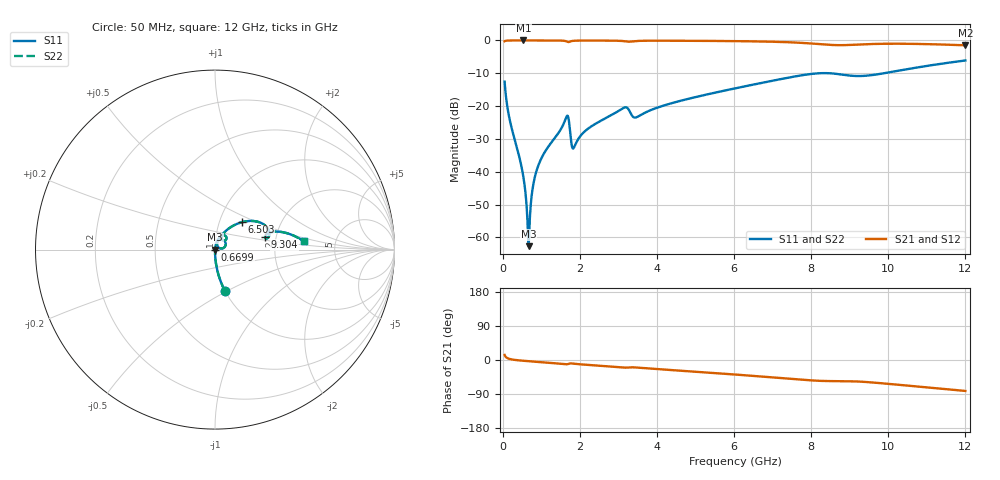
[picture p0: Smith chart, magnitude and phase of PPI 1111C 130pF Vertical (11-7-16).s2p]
# GHz S MA R 50
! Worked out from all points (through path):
!   1601 points, 50 MHz to 12 GHz, reference 50 ohm
!   highest |S21| = -0.01 dB at 535.5 MHz (marker M1); lowest = -1.5 dB at 12 GHz (marker M2)
!   group delay of S21, straight-line fit = 18.7 ps
!   lowest |S11| = -62.7 dB at 669.9 MHz (marker M3), VSWR 1.00, Z = 50.1 - j0.0112 ohm
!   |S11| at or under -10 dB: start of sweep to 8.202 GHz; 8.484 GHz to 9.885 GHz (1.401 GHz wide, 15.3 % of centre)
!   |S22| runs from -62.7 to -6.1 dB; largest |S21 - S12| = 0
!   S11 on the Smith chart (normalised r, x): 50 MHz: 1.00, -0.49; 669.9 MHz: 1.00, -0.00; 6.503 GHz: 1.28, +0.41; 9.304 GHz: 1.75, +0.27; 12 GHz: 2.91, +0.36
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0.05  0.2359 -76.5  0.9715 13.4  0.9715 13.4  0.2359 -76.5
0.1844375  0.06115 -87.0  0.9977 2.6  0.9977 2.6  0.06115 -87.0
0.5354688  0.008428 -87.5  0.9993 -2.0  0.9993 -2.0  0.008428 -87.5
0.6325625  0.002314 -74.9  0.9992 -2.8  0.9992 -2.8  0.002314 -74.9
0.6699063  0.0007361 -8.7  0.9992 -3.1  0.9992 -3.1  0.0007361 -8.7
0.70725  0.002094 65.5  0.9992 -3.4  0.9992 -3.4  0.002094 65.5
0.7744688  0.005451 77.7  0.9991 -4.0  0.9991 -4.0  0.005451 77.7
0.8416875  0.008675 80.1  0.9991 -4.5  0.9991 -4.5  0.008675 80.1
1.103094  0.02045 80.7  0.9987 -6.4  0.9987 -6.4  0.02045 80.7
1.655781  0.06891 52.5  0.9676 -11.3  0.9676 -11.3  0.06891 52.5
1.700594  0.06786 28.1  0.9459 -10.4  0.9459 -10.4  0.06786 28.1
1.827562  0.02258 42.5  0.9859 -9.6  0.9859 -9.6  0.02258 42.5
2.044156  0.03677 72.1  0.9952 -11.7  0.9952 -11.7  0.03677 72.1
3.142063  0.09442 57.7  0.9753 -20.0  0.9753 -20.0  0.09442 57.7
3.440812  0.06687 52.7  0.9775 -19.7  0.9775 -19.7  0.06687 52.7
4.038312  0.09602 63.0  0.9906 -24.3  0.9906 -24.3  0.09602 63.0
6.025  0.1862 49.8  0.9762 -38.3  0.9762 -38.3  0.1862 49.8
6.503  0.2127 45.7  0.9681 -42.0  0.9681 -42.0  0.2127 45.7
8.019156  0.3095 25.8  0.8969 -53.9  0.8969 -53.9  0.3095 25.8
9.303781  0.2874 14.1  0.8697 -57.3  0.8697 -57.3  0.2874 14.1
10.01331  0.3259 17.2  0.891 -63.0  0.891 -63.0  0.3259 17.2
12  0.4954 5.4  0.843 -81.7  0.843 -81.7  0.4954 5.4
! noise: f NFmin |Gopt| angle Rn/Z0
0.05  0.0003573  0.8609  0.3916  0.0005504
1.372  0.005021  0.7458  6.359  0.003959
2.701  0.009234  0.732  12.44  0.006792
4.031  0.01316  0.724  18.43  0.00923
5.36  0.01473  0.6849  24.04  0.008692
6.682  0.02506  0.7631  29.99  0.02006
8.012  0.06465  0.8849  35.99  0.1103
9.341  0.08964  0.9047  41.52  0.1804
10.67  0.06167  0.8507  46.57  0.07436
12  0.05359  0.8165  51.29  0.04976
